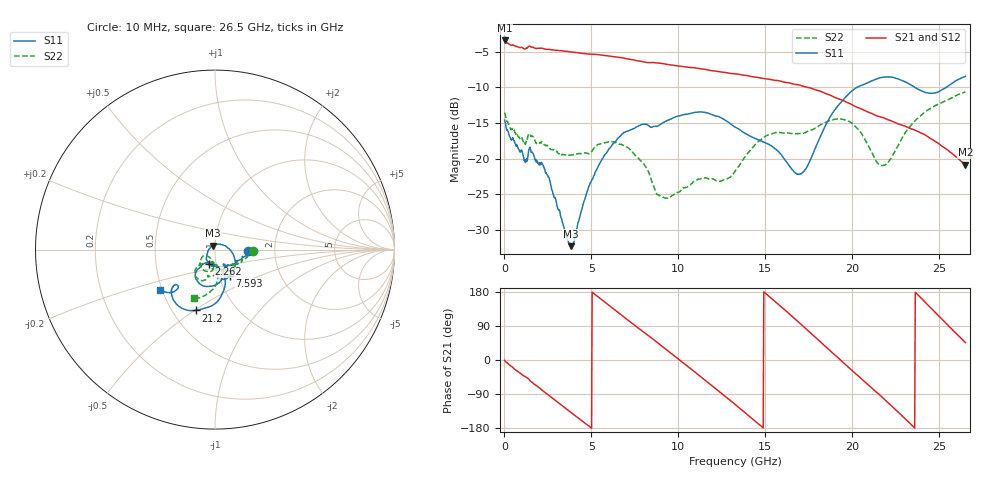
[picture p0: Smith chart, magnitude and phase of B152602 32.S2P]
!  2-Port S-parameters saved by WinCal
! VAR MeasName=S-Parameters (CALIBRATED_DATA) read from VNA (N5242A)
! VAR MeasDate=2016-1-5 16:30:48
! VAR NAME=B152602 32
! VAR FILENAME=B152602 32.S2P
! VAR DATE=2016-1-5 16:30:48
! VAR PHYS_PORTS=1,2
# Hz S DB R 50
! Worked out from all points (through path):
!   801 points, 10 MHz to 26.5 GHz, reference 50 ohm
!   highest |S21| = -3.40 dB at 10 MHz (marker M1); lowest = -20.9 dB at 26.5 GHz (marker M2)
!   group delay of S21, straight-line fit = 107 ps
!   lowest |S11| = -32.3 dB at 3.818 GHz (marker M3), VSWR 1.05, Z = 48.9 + j2.11 ohm
!   |S11| at or under -10 dB: start of sweep to 20.27 GHz; 23.6 GHz to 25.39 GHz (1.794 GHz wide, 7.32 % of centre)
!   |S22| runs from -25.6 to -10.6 dB; largest |S21 - S12| = 0.0028
!   S11 on the Smith chart (normalised r, x): 10 MHz: 1.46, -0.02; 2.262 GHz: 0.93, -0.15; 7.593 GHz: 1.13, -0.34; 21.2 GHz: 0.65, -0.51; 26.5 GHz: 0.49, -0.26
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1e7  -14.59 -1.9  -3.40 -0.8  -3.39 -0.7  -13.54 -1.7
1.168938e9  -20.15 -59.9  -4.54 -43.4  -4.54 -43.4  -17.76 -40.6
1.533175e9  -19.09 -74.8  -4.34 -56.9  -4.33 -56.9  -16.93 -51.8
2.26165e9  -21.19 -112.0  -4.56 -83.2  -4.56 -83.2  -17.99 -70.9
3.817938e9  -32.32 116.9  -5.01 -138.2  -5.00 -138.2  -19.50 -89.2
4.447075e9  -27.21 41.0  -5.20 -160.4  -5.20 -160.3  -19.29 -94.5
5.771575e9  -19.47 -15.6  -5.53 152.8  -5.52 152.8  -17.79 -109.2
6.731838e9  -16.63 -41.2  -5.82 118.3  -5.82 118.4  -18.01 -127.5
7.592762e9  -15.55 -60.0  -6.23 87.8  -6.20 87.9  -19.77 -142.2
8.851038e9  -15.41 -77.6  -6.56 44.0  -6.54 43.9  -25.13 -140.5
1.070534e10  -13.66 -99.5  -7.19 -22.7  -7.16 -22.7  -23.68 -107.3
1.196361e10  -13.84 -117.9  -7.66 -69.0  -7.63 -69.3  -22.84 -105.9
1.3255e10  -15.56 -129.7  -8.08 -117.0  -8.07 -117.1  -21.80 -85.6
1.517552e10  -17.98 -130.4  -8.84 169.4  -8.85 169.4  -16.68 -94.0
1.686426e10  -22.20 -107.7  -9.63 102.1  -9.63 102.0  -16.49 -105.4
1.769208e10  -19.58 -75.7  -10.17 67.5  -10.15 67.7  -15.93 -104.3
1.924836e10  -12.36 -79.4  -11.62 3.1  -11.60 3.0  -14.42 -118.4
2.1202e10  -8.99 -107.5  -13.76 -77.4  -13.74 -77.5  -19.55 -131.6
2.209604e10  -8.52 -121.7  -14.59 -114.5  -14.52 -114.7  -20.43 -97.6
2.335431e10  -9.61 -137.3  -15.78 -169.1  -15.75 -169.3  -15.37 -85.5
2.46457e10  -10.80 -135.8  -17.40 131.2  -17.38 130.9  -12.74 -95.4
2.65e10  -8.45 -143.6  -20.87 46.0  -20.84 45.7  -10.61 -113.3
